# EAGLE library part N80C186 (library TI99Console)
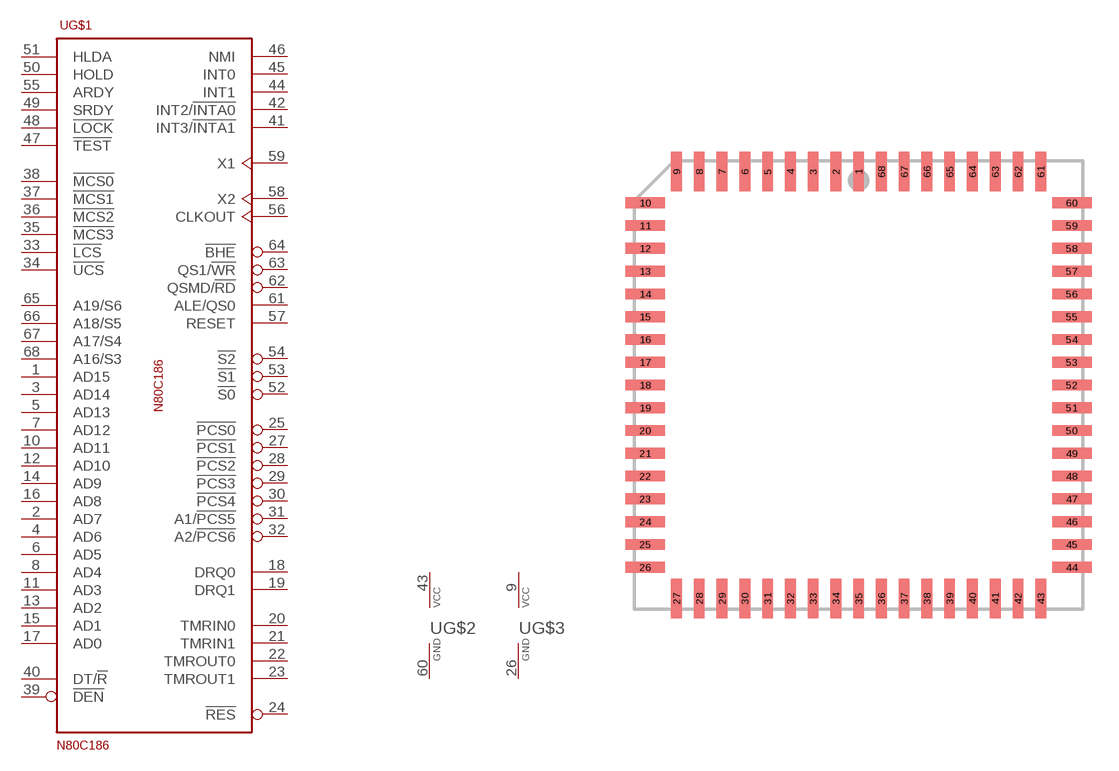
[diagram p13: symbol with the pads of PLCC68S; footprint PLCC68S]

Designator prefix -; gates G$1=N80C186 G$2=VCC-GND G$3=VCC-GND

## N80C186  [PLCC68S]
1  G$1:AD15
2  G$1:AD7
3  G$1:AD14
4  G$1:AD6
5  G$1:AD13
6  G$1:AD5
7  G$1:AD12
8  G$1:AD4
9  G$3:VCC  pwr
10  G$1:AD11
11  G$1:AD3
12  G$1:AD10
13  G$1:AD2
14  G$1:AD9
15  G$1:AD1
16  G$1:AD8
17  G$1:AD0
18  G$1:DRQ0  out
19  G$1:DRQ1  out
20  G$1:TMRIN0  out
21  G$1:TMRIN1  out
22  G$1:TMROUT0  out
23  G$1:TMROUT1  out
24  G$1:!RES  in
25  G$1:!PCS0  out
26  G$3:GND  pwr
27  G$1:!PCS1  out
28  G$1:!PCS2  out
29  G$1:!PCS3  out
30  G$1:!PCS4  out
31  G$1:A1/!PCS5  out
32  G$1:A2/!PCS6  out
33  G$1:!LCS
34  G$1:!UCS
35  G$1:!MCS3
36  G$1:!MCS2
37  G$1:!MCS1
38  G$1:!MCS0
39  G$1:!DEN
40  G$1:DT/!R
41  G$1:INT3/!INTA1  out
42  G$1:INT2/!INTA0  out
43  G$2:VCC  pwr
44  G$1:INT1  out
45  G$1:INT0  out
46  G$1:NMI  out
47  G$1:!TEST
48  G$1:!LOCK
49  G$1:SRDY
50  G$1:HOLD
51  G$1:HLDA
52  G$1:!S0  out
53  G$1:!S1  out
54  G$1:!S2  out
55  G$1:ARDY
56  G$1:CLKOUT  out
57  G$1:RESET  out
58  G$1:X2  in
59  G$1:X1  in
60  G$2:GND  pwr
61  G$1:ALE/QS0  out
62  G$1:QSMD/!RD  out
63  G$1:QS1/!WR  out
64  G$1:!BHE  out
65  G$1:A19/S6
66  G$1:A18/S5
67  G$1:A17/S4
68  G$1:A16/S3

## Footprint PLCC68S (pad centres in mm)
PLASTIC LEADED CHIP CARRIER square
smd 0.6 x 2.2: 1 0,11.9; 2 -1.27,11.9; 3 -2.54,11.9; 4 -3.81,11.9; 5 -5.08,11.9; 6 -6.35,11.9; 7 -7.62,11.9; 8 -8.89,11.9; 9 -10.16,11.9; 27 -10.16,-11.9; 28 -8.89,-11.9; 29 -7.62,-11.9; 30 -6.35,-11.9; 31 -5.08,-11.9; 32 -3.81,-11.9; 33 -2.54,-11.9; 34 -1.27,-11.9; 35 0,-11.9; 36 1.27,-11.9; 37 2.54,-11.9; 38 3.81,-11.9; 39 5.08,-11.9; 40 6.35,-11.9; 41 7.62,-11.9; 42 8.89,-11.9; 43 10.16,-11.9; 61 10.16,11.9; 62 8.89,11.9; 63 7.62,11.9; 64 6.35,11.9; 65 5.08,11.9; 66 3.81,11.9; 67 2.54,11.9; 68 1.27,11.9
smd 2.2 x 0.6: 10 -11.9,10.16; 11 -11.9,8.89; 12 -11.9,7.62; 13 -11.9,6.35; 14 -11.9,5.08; 15 -11.9,3.81; 16 -11.9,2.54; 17 -11.9,1.27; 18 -11.9,0; 19 -11.9,-1.27; 20 -11.9,-2.54; 21 -11.9,-3.81; 22 -11.9,-5.08; 23 -11.9,-6.35; 24 -11.9,-7.62; 25 -11.9,-8.89; 26 -11.9,-10.16; 44 11.9,-10.16; 45 11.9,-8.89; 46 11.9,-7.62; 47 11.9,-6.35; 48 11.9,-5.08; 49 11.9,-3.81; 50 11.9,-2.54; 51 11.9,-1.27; 52 11.9,0; 53 11.9,1.27; 54 11.9,2.54; 55 11.9,3.81; 56 11.9,5.08; 57 11.9,6.35; 58 11.9,7.62; 59 11.9,8.89; 60 11.9,10.16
